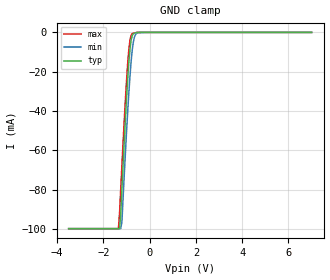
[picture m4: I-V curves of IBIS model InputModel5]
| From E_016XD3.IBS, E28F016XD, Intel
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|**********************Input Model 5*****************************************
[Model]   InputModel5
Model_type   Input
|   for pin29(NC), pin30(NC)
Vinl = 0.8V
Vinh = 2.0V
| Variable   typ   min   max
C_comp   5.61p   NA   7.6p
[Voltage Range]   3.3V   3.0V   3.6V
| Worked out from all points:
|   GND clamp passes 1 mA (typ) near -0.72 V on its own axis
[GND_clamp]
|Voltage I(typ)   I(min)   I(max)
-3.5V     -99.85mA   -99.84mA   -99.85mA
-1.35V    -99.85mA   -99.84mA   -99.85mA
-1.3V     -99.85mA   -99.84mA   -91.85mA
-1.25V    -92.41mA   -99.84mA   -79.73mA
-1.2V     -79.97mA   -96.6mA    -67.96mA
-1.05V    -44.56mA   -61.78mA   -34.68mA
-950mV    -23.88mA   -40.48mA   -15.91mA
-850mV    -8.536mA   -22.25mA   -3.899mA
-750mV    -1.559mA   -8.689mA   -616.5uA
-650mV    -317.1uA   -2.102mA   -225.6uA
-500mV    0A         -132.3uA   0A
7V        0A         0A         0A
[POWER_clamp]
| Input buffer circuits of this product do not intrinsically
| require a [POWER_clamp] definition.  This zero current
| [POWER_clamp] is provided for compatibility with some ibis
| parsers.
|Voltage  I(typ)   I(min)   I(max)
-3.3V     0A         0A         0A
-3V       0A         0A         0A
6.3V      0A         0A         0A
6.6V      0A         0A         0A
